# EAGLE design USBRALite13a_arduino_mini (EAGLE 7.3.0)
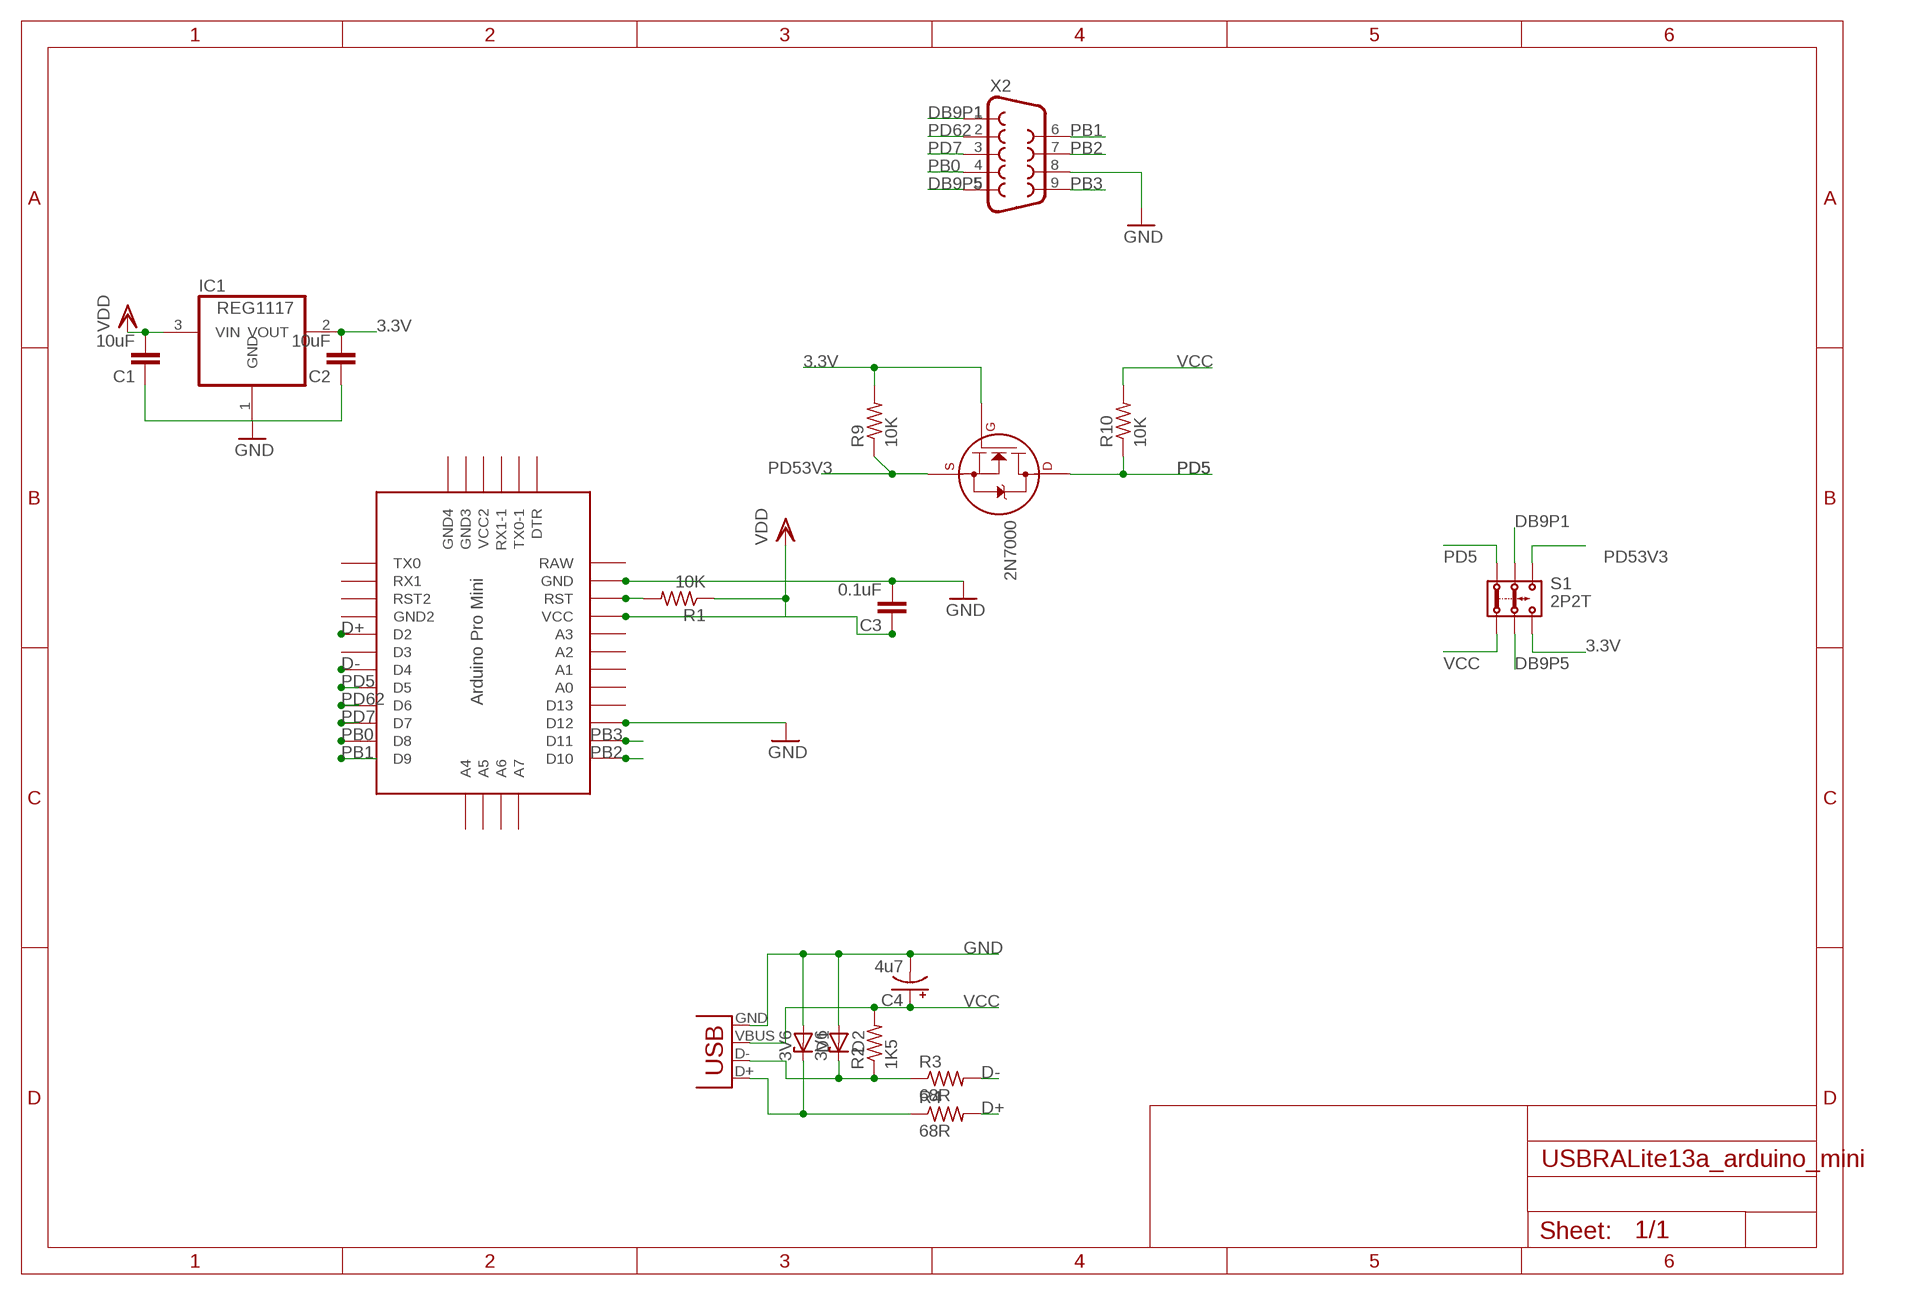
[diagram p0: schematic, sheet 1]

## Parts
2N7000  2N7000_TO92  [TO-92]
C1  10uF  C-EUC0603  [C0603]
C2  10uF  C-EUC0603  [C0603]
C3  0.1uF  C-EUC0603  [C0603]
C4  4u7  CPOL-USE2.5-6  [E2,5-6]
D1  3V6  ZENER-DIODEZD-5  [ZDIO-5]
D2  3V6  ZENER-DIODEZD-5  [ZDIO-5]
IC1  REG1117  [SOT223]
R1  10K  R-US_R0603  [R0603]
R2  1K5  R-US_R0603  [R0603]
R3  68R  R-US_R0603  [R0603]
R4  68R  R-US_R0603  [R0603]
R9  10K  R-US_R0603  [R0603]
R10  10K  R-US_R0603  [R0603]
S1  2P2T  [2P2T]
U$1  PRO-MINI  [PRO-MINI]
X1  USBPTH  [USB-B-PTH]
X2  DB9MALE  [DB9_MALE]

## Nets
3.3V: 2N7000.2(G) C2.2 IC1.2(VOUT) R9.2 S1.3.2
D+: R4.2 U$1.D2
D-: R3.2 U$1.D4
DB9P1: S1.2.1 X2.1
DB9P5: S1.2.2 X2.5
GND: C1.1 C2.1 C3.2 C4.- D1.A D2.A IC1.1(GND) U$1.D12 U$1.GND X1.GND X2.8
N$1: R1.2 U$1.RST
N$8: D1.C R4.1 X1.D+
N$9: D2.C R2.1 R3.1 X1.D-
PB0: U$1.D8 X2.4
PB1: U$1.D9 X2.6
PB2: U$1.D10 X2.7
PB3: U$1.D11 X2.9
PD5: 2N7000.3(D) R10.1 S1.1.1 U$1.D5
PD7: U$1.D7 X2.3
PD53V3: 2N7000.1(S) R9.1 S1.3.1
PD62: U$1.D6 X2.2
VCC: C3.1 C4.+ R1.1 R2.2 R10.2 S1.1.2 X1.VBUS ; supply symbol labelled VDD
VDD: C1.2 IC1.3(VIN)
Unconnected: U$1.A0 U$1.A1 U$1.A2 U$1.A3 U$1.A4 U$1.A5 U$1.A6 U$1.A7 U$1.D3 U$1.D13 U$1.DTR U$1.GND1(GND2) U$1.GND2(GND4) U$1.GND3 U$1.RST1(RST2) U$1.RX1 U$1.RX1-1 U$1.TX0 U$1.TX0-1 U$1.VCC U$1.VCC1(VCC2)

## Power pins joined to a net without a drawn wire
RAW: U$1.RAW

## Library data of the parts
2N7000 = transistors:2N700*: 2N7000, 2N7002, NDS7002A N-channel enhancement mode MOSFET
C1-C3 = rcl:C-EU: CAPACITOR, European symbol
C4 = adafruit:CPOL-US: POLARIZED CAPACITOR, American symbol
D1 D2 = diode:ZENER-DIODE: Z-Diode
IC1 = burr-brown:REG1117: 800mA and 1A Low Dropout (LDO) Positive Regulator 1.8V, 2.5V, 2.85V, 3.3V, 5V, and Adj; MPN: REG1117; OC_FARNELL: 1097566; OC_NEWARK: 14P6981
R1-R4 R9 R10 = adafruit:R-US_: RESISTOR, American symbol
S1 = Itead_BP_110825:2P2T: BAS011
U$1 = Arduino-clone:PRO-MINI: Arduion Pro Mini Clone V1.0 www.betemcu.cu
X1 = SparkFun:USB: USB Connectors USB-B-PTH is fully proven SKU : PRT-00139 USB-miniB is fully proven SKU : PRT-00587 USB-A-PCB is untested. USB-A-H is throughly reviewed, but untested. Spark Fun Electronics SKU : PRT-00437 USB-B-SMT is throughly reviewed, but untested. Needs silkscreen touching up. USB-A-S has not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
X2 = SparkFun:DB9: DB9 Connector Standard DB9 (D-Sub 9) serial connector. Can be used for CAN bus as well as RS485 and RS232. Footprint production proven. Spark Fun Electronics SKU : PRT-00429

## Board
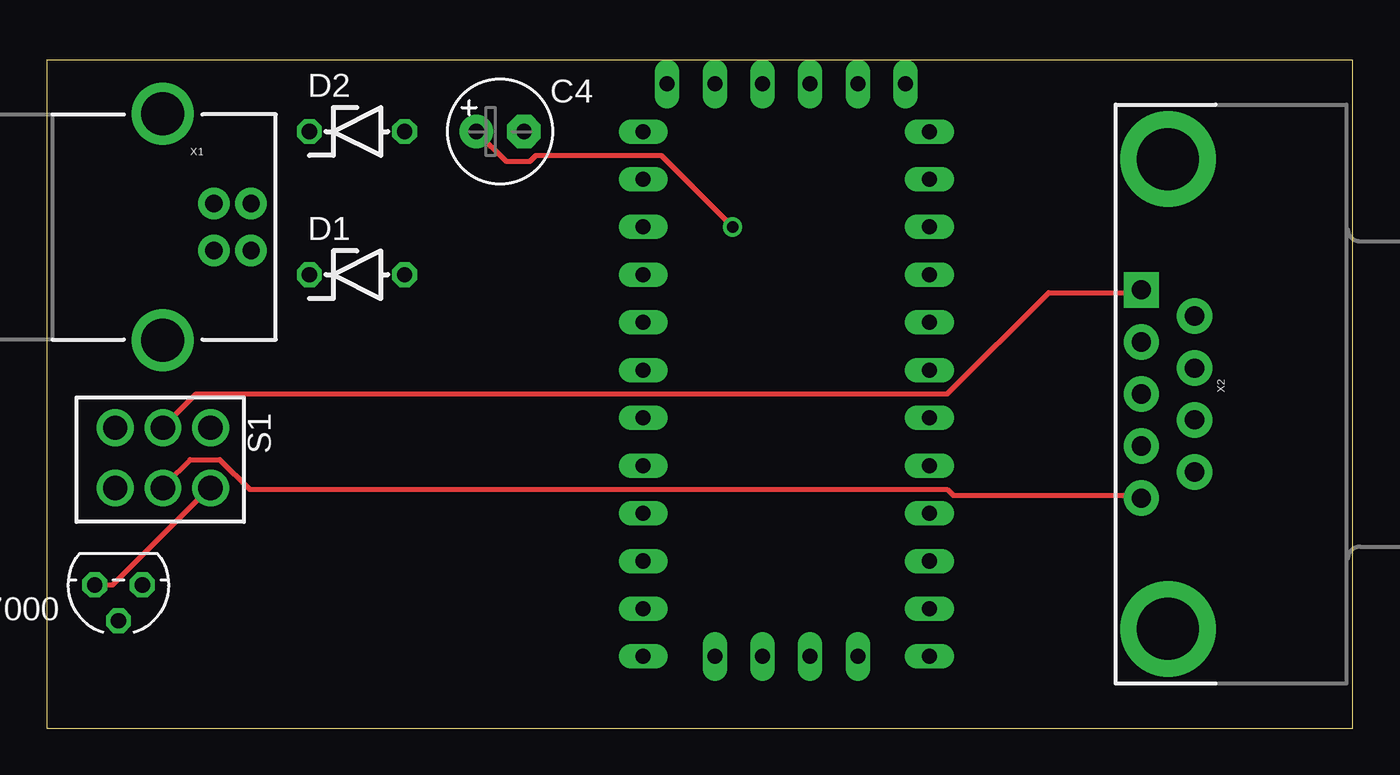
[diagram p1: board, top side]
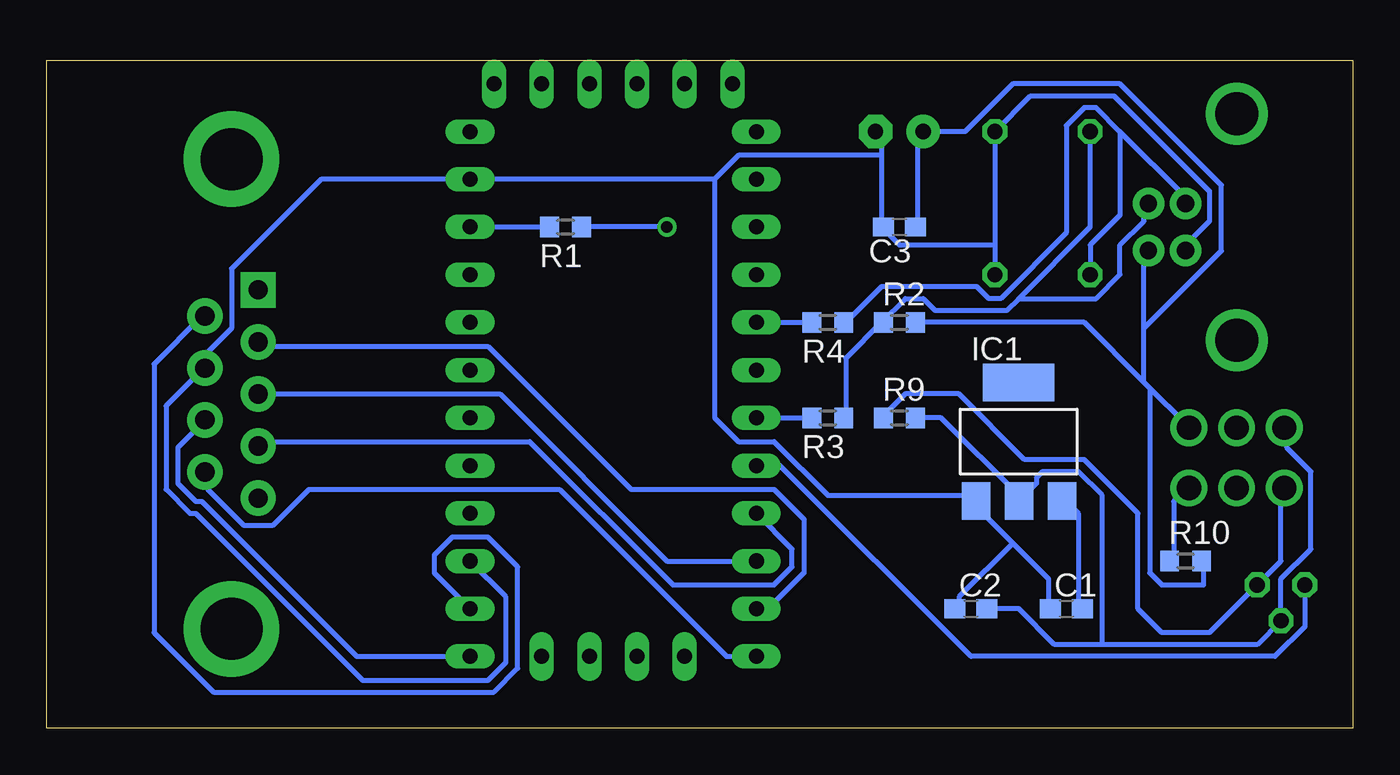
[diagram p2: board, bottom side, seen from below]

Size 69.52 x 35.55 mm. Coordinates in mm from the lower left corner, seen from the top.
Outline: 0,0 69.52,0 69.52,35.55 0,35.55 0,0
Copper layers (1*16): Top 0.035mm / dielectric 1.5mm / Bottom 0.035mm
Design rules "default *": minimum track width 10mil, minimum drill 24mil, track to track 12mil, track to pad 12mil, pad to pad 12mil, via to via 12mil, smd to smd 12mil, copper to edge 40mil, drill to drill 8mil, minimum pad ring 10mil, minimum via ring 8mil, stop-mask expansion 4mil, vias tented up to drill 0mil, thermal gap 10mil

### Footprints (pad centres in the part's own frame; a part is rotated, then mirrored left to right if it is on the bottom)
TO-92 = drill 0.813 octagon: 1 -1.27,0; 2 0,1.905; 3 1.27,0
C0603 = smd 1.1 x 1: 1 -0.85,0; 2 0.85,0
E2,5-6 = drill 0.813 pad 1.778: + -1.27,0 | drill 0.813 pad 1.778 octagon: - 1.27,0
ZDIO-5 = drill 0.813 octagon: A 2.54,0; C -2.54,0
SOT223 = smd 1.499 x 2.007: 1 -2.261,-3.15; 2 0.025,-3.15; 3 2.311,-3.15 | smd 3.81 x 2.007: 4 0,3.15
R0603 = smd 1 x 1.1: 1 -0.85,0; 2 0.85,0
2P2T = drill 1.3 pad 1.93: 1.1 -3.635,-0.085; 1.2 -3.635,-3.285; 2.1 -1.095,-0.085; 2.2 -1.095,-3.285; 3.1 1.445,-0.085; 3.2 1.445,-3.285
PRO-MINI = drill 0.8 long: A0 8.89,8.89; A1 8.89,11.43; A2 8.89,13.97; A3 8.89,16.51; A4 -2.54,-1.27; A5 0,-1.27; A6 2.54,-1.27; A7 5.08,-1.27; D2 -6.35,16.51; D3 -6.35,13.97; D4 -6.35,11.43; D5 -6.35,8.89; D6 -6.35,6.35; D7 -6.35,3.81; D8 -6.35,1.27; D9 -6.35,-1.27; D10 8.89,-1.27; D11 8.89,1.27; D12 8.89,3.81; D13 8.89,6.35; DTR 7.62,29.21; GND 8.89,24.13; GND1 -6.35,19.05; GND2 -5.08,29.21; GND3 -2.54,29.21; RAW 8.89,26.67; RST 8.89,21.59; RST1 -6.35,21.59; RX1 -6.35,24.13; RX1-1 2.54,29.21; TX0 -6.35,26.67; TX0-1 5.08,29.21; VCC 8.89,19.05; VCC1 0,29.21
USB-B-PTH = drill 0.914 pad 1.676: D+ 0,1.25; D- 1.981,1.25; GND 0,-1.25; VBUS 1.981,-1.25 | drill 2.286: S1 -2.718,-6.02; S2 -2.718,6.02
DB9_MALE = drill 1.016 pad 1.88: 1 5.54,-1.42; 2 2.77,-1.42; 3 0,-1.42; 4 -2.77,-1.42; 6 4.15,1.42; 7 1.38,1.42; 8 -1.38,1.42; 9 -4.15,1.42 | drill 1.016 pad 1.88 square: 5 -5.54,-1.42 | drill 3.302 pad 5.08: G1 -12.5,0; G2 12.5,0

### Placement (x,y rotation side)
2N7000  3.81,7.62 180 top
C1  15.24,6.35 0 bottom
C2  20.32,6.35 0 bottom
C3  24.13,26.67 180 bottom
C4  24.13,31.75 0 top
D1  16.51,24.13 0 top
D2  16.51,31.75 0 top
IC1  17.78,15.24 0 bottom
R1  41.91,26.67 180 bottom
R2  24.13,21.59 0 bottom
R3  27.94,16.51 180 bottom
R4  27.94,21.59 180 bottom
R9  24.13,16.51 0 bottom
R10  8.89,8.89 0 bottom
S1  5.08,12.7 180 top
U$1  38.1,5.08 0 top
X1  8.89,26.67 0 top
X2  59.69,17.78 270 top

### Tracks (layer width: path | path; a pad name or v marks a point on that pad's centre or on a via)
3.3V
  Bottom 0.254: R9.2 21.91,16.51 17.78,12.38 IC1.2 16.83,13.02 16.83,13.33 16.51,13.65 14.61,13.65 13.34,12.38 13.34,4.45 | C2.2 17.78,6.35 15.88,4.45 13.34,4.45 | 13.34,4.45 5.08,4.45 2N7000.2 3.81,7.94 2.22,9.52 2.22,13.65 3.49,14.92 3.49,15.88 S1.3.2
D+
  Bottom 0.254: U$1.D2 R4.2
D-
  Bottom 0.254: U$1.D4 R3.2
DB9P1
  Top 0.254: X2.1 58.1,12.38 48.26,12.38 47.94,12.7 10.79,12.7 9.21,14.29 7.62,14.29 6.35,13.02 S1.2.1
DB9P5
  Top 0.254: X2.5 58.1,23.18 53.34,23.18 47.94,17.78 7.94,17.78 6.35,16.19 S1.2.2
GND
  Bottom 0.254: U$1.D12 45.09,6.98 45.09,3.49 46.04,2.54 52.7,2.54 61.59,11.43 61.91,11.43 63.18,12.7 63.18,17.14 61.28,19.05 X2.8 60.96,19.37 60.96,20 59.69,21.27 59.69,24.45 54.93,29.21 U$1.GND 33.97,29.21 | 19.05,25.72 D2.A 17.14,33.66 12.7,33.66 7.62,28.58 7.62,26.99 8.89,25.72 X1.GND | 19.05,25.72 D1.A | 18.1,9.84 20.32,12.06 IC1.1 20.32,12.38 27.94,12.38 30.8,15.24 32.7,15.24 33.97,16.51 33.97,29.21 | 18.1,9.84 16.19,7.94 16.19,6.35 C1.1 | 18.1,9.84 20.95,6.98 20.95,6.35 C2.1 | 25.08,30.48 25.08,31.43 C4.- | 25.08,30.48 25.08,26.67 | 33.97,29.21 32.7,30.48 25.08,30.48 | 19.05,25.72 24.13,25.72 25.08,26.67 | 25.08,26.67 C3.2
N$1
  Bottom 0.254: U$1.RST R1.2
N$8
  Bottom 0.254: 12.38,31.75 8.89,28.26 X1.D+ | 12.38,31.75 13.65,33.02 14.29,33.02 15.24,32.07 15.24,26.35 18.73,22.86 19.37,22.86 20,23.49 25.08,23.49 26.99,21.59 R4.1 | D1.C 13.97,25.72 12.38,27.3 12.38,31.75
N$9
  Bottom 0.254: 25.08,21.59 26.99,19.69 26.99,16.51 R3.1 | D2.C 13.97,26.67 17.78,22.86 | 17.78,22.86 18.41,22.22 22.23,22.22 22.86,22.86 23.81,22.86 25.08,21.59 | 25.08,21.59 R2.1 | 17.78,22.86 13.65,22.86 12.38,24.13 12.38,25.72 11.11,26.99 11.11,27.62 X1.D-
PB0
  Bottom 0.254: U$1.D8 31.11,6.35 29.21,8.25 29.21,11.11 30.8,12.7 38.42,12.7 46.04,20.32 58.1,20.32 X2.4
PB1
  Bottom 0.254: U$1.D9 33.34,3.81 42.23,12.7 55.56,12.7 57.47,10.79 59.05,10.79 60.96,12.7 60.96,13.33 X2.6
PB2
  Bottom 0.254: U$1.D10 53.02,3.81 61.28,12.06 61.59,12.06 62.55,13.02 62.55,14.92 61.28,16.19 X2.7
PB3
  Bottom 0.254: U$1.D11 48.9,8.25 48.9,9.21 47.94,10.16 46.04,10.16 44.45,8.57 44.45,3.17 45.72,1.9 60.64,1.9 63.82,5.08 63.82,19.37 61.28,21.91 X2.9
PD5
  Top 0.254: 2N7000.3 3.49,7.62 8.57,12.7 S1.1.1
  Bottom 0.254: R10.1 9.53,8.89 9.53,12.06 8.89,12.7 S1.1.1 | U$1.D5 30.48,13.97 20.32,3.81 4.13,3.81 2.54,5.4 2N7000.3
PD7
  Bottom 0.254: U$1.D7 36.51,8.89 45.4,17.78 X2.3
PD53V3
  Bottom 0.254: R9.1 24.77,16.51 24.77,16.83 23.81,17.78 20.95,17.78 17.46,14.29 14.29,14.29 11.43,11.43 11.43,6.35 10.16,5.08 7.62,5.08 2N7000.1 3.81,8.89 3.81,12.7 S1.3.1
PD62
  Bottom 0.254: U$1.D6 29.84,9.52 29.84,8.57 30.8,7.62 36.2,7.62 43.81,15.24 58.1,15.24 X2.2
VCC  (via drill 0.61)
  Top 0.254: v36.51,26.67 32.7,30.48 26.04,30.48 25.72,30.16 24.45,30.16 C4.+
  Bottom 0.254: C3.1 23.18,26.67 23.18,31.43 C4.+ 20.64,31.75 18.1,34.29 12.38,34.29 6.99,28.89 6.99,25.4 11.11,21.27 | R10.2 7.94,8.89 7.94,7.62 10.16,7.62 10.79,8.25 10.79,18.1 | R2.2 14.29,21.59 11.11,18.41 | 10.79,18.1 8.89,16.19 S1.1.2 | 10.79,18.1 11.11,18.41 | 11.11,18.41 11.11,21.27 | 11.11,21.27 11.11,25.4 X1.VBUS | v36.51,26.67 R1.1
VDD
  Bottom 0.254: C1.2 14.61,6.35 14.61,11.43 15.24,12.06 IC1.3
